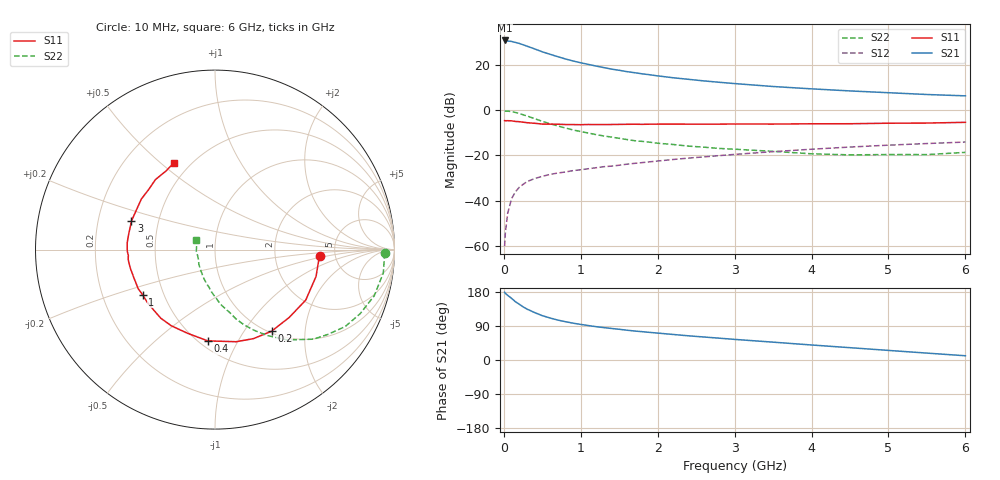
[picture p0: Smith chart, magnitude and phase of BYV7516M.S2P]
! SIEMENS Small Signal Semiconductors
! BFY420
! Si NPN RF SIEGET Grounded Emitter Transistor in MICRO-X
! VCE = 0.75 V  IC = 16 mA
! Common Emitter S-Parameters:  October  1996
# GHz  S  MA  R  50
!  f  S11  S21  S12  S22
! GHz  MAG  ANG  MAG  ANG  MAG  ANG  MAG  ANG
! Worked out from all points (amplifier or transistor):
!   36 points, 10 MHz to 6 GHz, reference 50 ohm
!   highest |S21| = 30.7 dB at 10 MHz (marker M1)
!   |S21| within 3 dB of that: start of sweep to 341 MHz
!   unconditionally stable (mu >= 1): 1.924 GHz to end of sweep
!   at 250 MHz: K = 0.27, MSG = 30.8 dB, |S12| = -32.8 dB
!   at 1.4 GHz: K = 0.90, MSG = 21.4 dB, |S12| = -24.7 dB
!   at 6 GHz: K = 1.10, MAG = 8.2 dB, |S12| = -14.1 dB
!   S11 on the Smith chart (normalised r, x): 10 MHz: 3.78, -0.41; 200 MHz: 1.03, -1.35; 400 MHz: 0.55, -0.76; 1 GHz: 0.38, -0.25; 3 GHz: 0.35, +0.15; 6 GHz: 0.41, +0.56
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0.01  0.586 -3.5  34.13 178.9  0.001 96.0  0.9464 -1.2
0.02  0.5806 -6.5  33.85 175.9  0.002 78.3  0.9446 -2.8
0.05  0.5825 -14.9  33.23 170.7  0.0053 79.8  0.9467 -7.9
0.1  0.5786 -29.1  32.42 162.8  0.0111 78.6  0.9236 -16.2
0.15  0.5602 -42.4  30.88 153.9  0.0157 72.4  0.8842 -23.8
0.2  0.5533 -55.3  29.38 147.3  0.0198 68.7  0.8425 -30.6
0.25  0.5404 -66.6  27.46 140.2  0.023 64.0  0.7866 -36.9
0.3  0.5266 -77.1  25.6 134.5  0.0264 61.2  0.7415 -42.3
0.4  0.5101 -94.5  22.25 125.2  0.0309 56.2  0.645 -51.3
0.5  0.4907 -108.1  19.18 117.0  0.0346 53.4  0.5634 -58.4
0.6  0.4893 -119.8  16.93 110.9  0.0381 51.4  0.4992 -64.2
0.7  0.4872 -128.3  15.02 105.4  0.0409 50.2  0.4471 -69.1
0.8  0.4794 -136.1  13.36 101.1  0.0431 49.3  0.4016 -73.3
1  0.4754 -148.1  10.99 93.9  0.0483 49.6  0.3353 -79.9
1.1  0.4801 -153.0  10.11 90.8  0.0509 49.5  0.3108 -83.5
1.6  0.4849 -170.9  7.022 78.6  0.0641 49.4  0.2237 -96.9
2.2  0.4905 175.5  5.144 67.4  0.0813 48.3  0.1741 -110.4
3  0.492 161.1  3.829 54.4  0.1053 44.5  0.137 -126.1
3.5  0.4905 153.0  3.299 47.1  0.121 41.3  0.1228 -136.9
4.5  0.4989 137.5  2.637 32.5  0.1529 33.1  0.1028 -158.6
5.5  0.5163 121.8  2.199 18.2  0.1827 23.4  0.1043 168.0
6  0.5359 115.2  2.053 11.2  0.197 18.4  0.1167 152.9
